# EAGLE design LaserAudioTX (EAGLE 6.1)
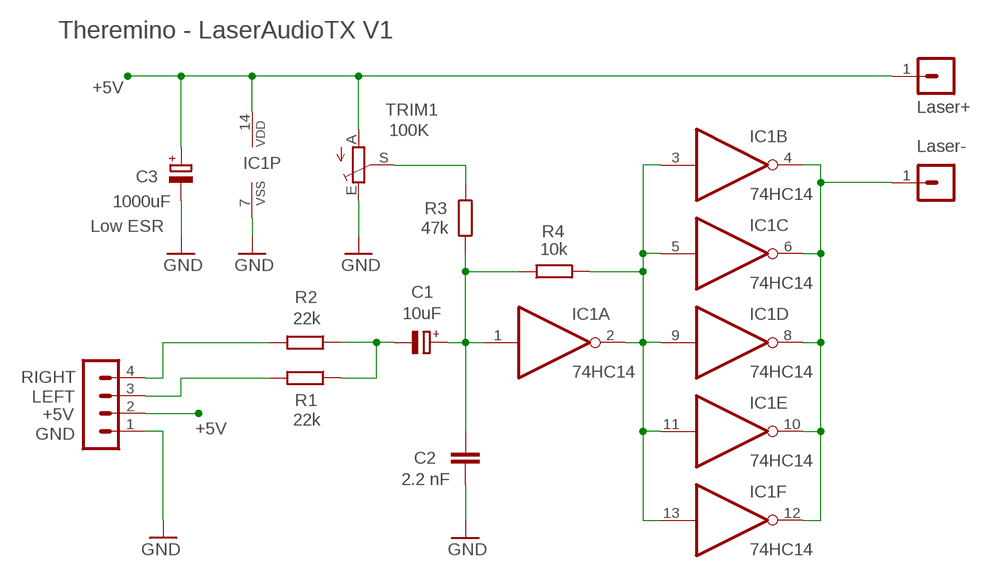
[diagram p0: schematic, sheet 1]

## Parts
C1  10uF  CPOL-EUE2-5B  [E2-5B]
C2  2.2 nF  C5/2.5  [C5B2.5]
C3  1000uF  CPOL-EUE10-22-R  [E10-22-R]
IC1  74HC14  40106DIL  [DIL14]
R1  22k  R-EU_0204/7  [0204/7]
R2  22k  R-EU_0204/7  [0204/7]
R3  47k  R-EU_0204/7  [0204/7]
R4  10k  R-EU_0204/5  [0204/5]
SV2  Laser-  MA01-1  [MA01-1]
SV3  Laser+  MA01-1  [MA01-1]
SV5  PWM  MA04-11  [MA04-1]
TRIM1  100K  TRIMMERTRIM_2H  [TRIM_2H]

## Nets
+5V: C3.V+ IC1.14(P:VDD) SV3.1 SV5.2 TRIM1.A
GND: C2.2 C3.V- IC1.7(P:VSS) SV5.1 TRIM1.E
N$1: C1.V- R1.1 R2.1
N$2: IC1.2(A:O) IC1.3(B:I) IC1.5(C:I) IC1.9(D:I) IC1.11(E:I) IC1.13(F:I) R4.2
N$3: IC1.4(B:O) IC1.6(C:O) IC1.8(D:O) IC1.10(E:O) IC1.12(F:O) SV2.1
N$4: C1.V+ C2.1 IC1.1(A:I) R3.2 R4.1
N$6: R1.2 SV5.3
N$7: R2.2 SV5.4
N$8: R3.1 TRIM1.S

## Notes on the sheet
- Theremino - LaserAudioTX V1

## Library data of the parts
C1 = 00-LIVIO:CPOL-EU: POLARIZED CAPACITOR, European symbol
C2 = 00-LIVIO:C: CAPACITOR
C3 = 00-LIVIO:CPOL-EU: POLARIZED CAPACITOR, European symbol; 1: Low ESR
IC1 = 00-LIVIO:40106: Hex SCHMITT TRIGGER 40106 74C14
R1-R4 = 00-LIVIO:R-EU_: RESISTOR, European symbol
SV2 SV3 = 03-con-lstb-M:MA01-1: PIN HEADER
SV5 = 03-con-lstb-M:MA04-1: PIN HEADER; 5V: +5V; GND: GND; LEFT: L; RIGHT: R
TRIM1 = 00-LIVIO:TRIMMER: Horizzontal and Vertical trimmers

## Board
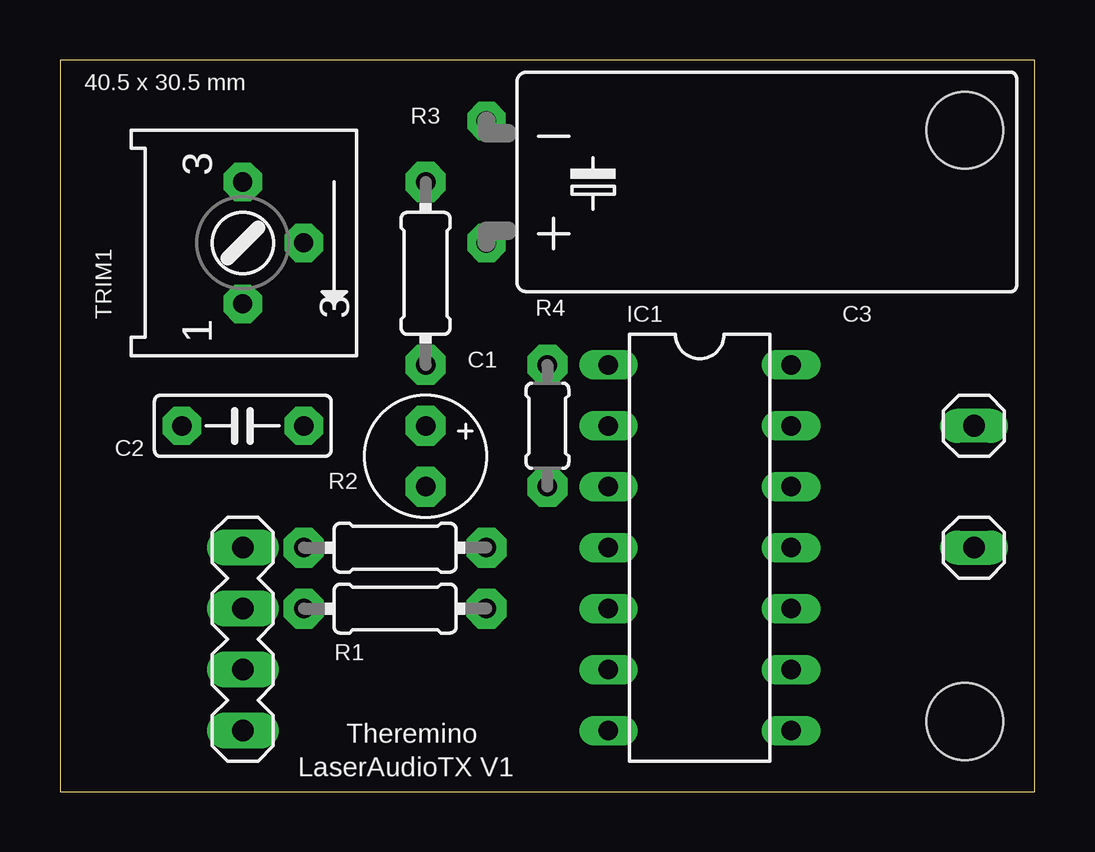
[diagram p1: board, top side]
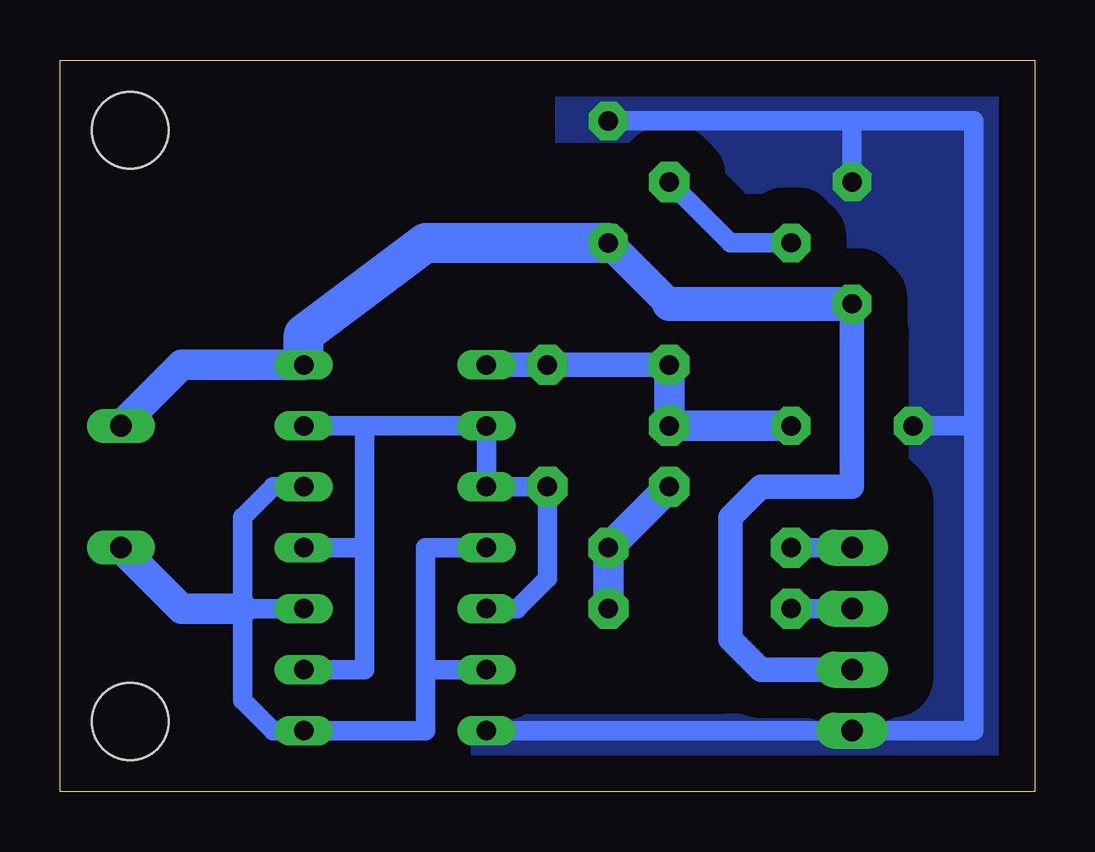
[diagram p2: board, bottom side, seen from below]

Size 40.64 x 30.48 mm. Coordinates in mm from the lower left corner, seen from the top.
Outline: 0,0 40.64,0 40.64,30.48 0,30.48 0,0
Copper layers (1*16): Top 0.035mm / dielectric 1.5mm / Bottom 0.035mm
Design rules: minimum track width 10mil, minimum drill 23mil, track to track 23mil, track to pad 23mil, pad to pad 23mil, via to via 23mil, smd to smd 23mil, copper to edge 23mil, drill to drill 8mil, minimum pad ring 5mil, minimum via ring 8mil, stop-mask expansion 4mil, vias tented up to drill 0mil, thermal gap 35mil
Holes 3.2 mm at 37.72,27.56 37.72,2.92
bRestrict: 6 lines

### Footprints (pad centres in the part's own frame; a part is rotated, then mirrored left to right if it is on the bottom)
E2-5B = drill 0.813 pad 1.676 octagon: V+ -1.27,0; V- 1.27,0
C5B2.5 = drill 0.813 pad 1.6 octagon: 1 -2.54,0; 2 2.54,0
E10-22-R = drill 0.813 pad 1.6 octagon: V+ 2.54,0; V- -2.54,0
DIL14 = drill 0.813 long: 1 -7.62,-3.81; 2 -5.08,-3.81; 3 -2.54,-3.81; 4 0,-3.81; 5 2.54,-3.81; 6 5.08,-3.81; 7 7.62,-3.81; 8 7.62,3.81; 9 5.08,3.81; 10 2.54,3.81; 11 0,3.81; 12 -2.54,3.81; 13 -5.08,3.81; 14 -7.62,3.81
0204/7 = drill 0.813 pad 1.676 octagon: 1 -3.81,0; 2 3.81,0
0204/5 = drill 0.813 pad 1.676 octagon: 1 -2.54,0; 2 2.54,0
MA01-1 = drill 0.9 pad 1.422 long: 1 0,0
MA04-1 = drill 0.9 pad 1.5 long: 1 -3.81,0; 2 -1.27,0; 3 1.27,0; 4 3.81,0
TRIM_2H = drill 0.8 pad 1.6 octagon: A 2.54,0; E -2.54,0; S 0,2.54

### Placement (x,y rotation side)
C1  15.24,13.97 270 top
C2  7.62,15.24 180 top
C3  17.78,25.4 270 top
IC1  26.67,10.16 270 top
R1  13.97,7.62 180 top
R2  13.97,10.16 180 top
R3  15.24,21.59 270 top
R4  20.32,15.24 270 top
SV2  38.1,10.16 270 top
SV3  38.1,15.24 90 top
SV5  7.62,6.35 90 top
TRIM1  7.62,22.86 270 top

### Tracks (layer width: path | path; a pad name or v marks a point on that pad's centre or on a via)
+5V
  Bottom 1.016: SV5.2 11.43,5.08 12.7,6.35 12.7,11.43 11.43,12.7 7.62,12.7 TRIM1.A
  Bottom 1.27: SV3.1 35.56,17.78 IC1.14 30.48,18.16 | C3.V+ 15.24,20.32
  Bottom 1.422: 15.24,20.32 TRIM1.A
  Bottom 1.676: 30.48,18.16 30.48,19.05 25.4,22.86 C3.V+
GND
  Bottom 0.813: 2.54,15.24 2.54,2.54 SV5.1 IC1.7 | C2.2 2.54,15.24 | 2.54,15.24 2.54,27.94 7.62,27.94 | 7.62,27.94 C3.V- | 7.62,27.94 TRIM1.E
  pour Bottom (isolate 1.5, no thermals): -1,-1 41.64,-1 41.64,31.48 -1,31.48
N$1
  Bottom 1.27: C1.V- R2.1 R1.1
N$2
  Bottom 0.813: IC1.13 27.94,15.24 | 27.94,15.24 27.94,10.16 | IC1.11 27.94,10.16 | 27.94,10.16 27.94,5.08 IC1.9 | IC1.5 21.59,7.62 20.32,8.89 R4.2 IC1.3 IC1.2 27.94,15.24
N$3
  Bottom 0.813: IC1.12 31.75,12.7 33.02,11.43 33.02,7.62 | IC1.10 33.02,7.62 | 33.02,7.62 33.02,3.81 31.75,2.54 IC1.8 25.4,2.54 25.4,5.08 | IC1.6 25.4,5.08 | IC1.4 25.4,10.16 25.4,5.08
  Bottom 1.27: 33.02,7.62 35.56,7.62 SV2.1
N$4
  Bottom 1.016: R3.2 R4.1 IC1.1
  Bottom 1.27: C2.1 C1.V+ R3.2
N$6
  Bottom 0.813: SV5.3 R1.2
N$7
  Bottom 0.813: R2.2 SV5.4
N$8
  Bottom 0.813: TRIM1.S 12.7,22.86 R3.1

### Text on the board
tNames: 40.5 x 30.5 mm | Theremino | LaserAudioTX V1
